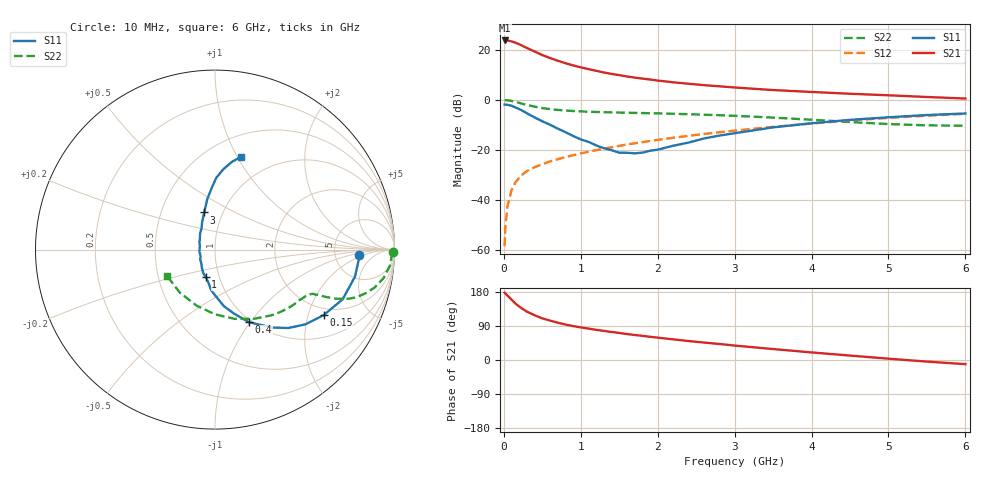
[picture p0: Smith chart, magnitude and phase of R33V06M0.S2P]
! SIEMENS Small Signal Semiconductors
! BFR181
! Si NPN RF Bipolar Junction Transistor in SOT23
! VCE = 3 V  IC = 6 mA
! Common Emitter S-Parameters:  May  1996
# GHz  S  MA  R  50
!  f  S11  S21  S12  S22
! GHz  MAG  ANG  MAG  ANG  MAG  ANG  MAG  ANG
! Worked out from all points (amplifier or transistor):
!   36 points, 10 MHz to 6 GHz, reference 50 ohm
!   highest |S21| = 23.7 dB at 10 MHz (marker M1)
!   |S21| within 3 dB of that: start of sweep to 300.1 MHz
!   unconditionally stable (mu >= 1): 993.5 MHz to 2.812 GHz
!   at 250 MHz: K = 0.47, MSG = 25.5 dB, |S12| = -29.6 dB
!   at 1.4 GHz: K = 1.05, MAG = 13.3 dB, |S12| = -18.9 dB
!   at 6 GHz: K = 0.86, MSG = 3.1 dB, |S12| = -5.6 dB
!   S11 on the Smith chart (normalised r, x): 10 MHz: 8.97, -1.65; 150 MHz: 1.73, -2.53; 400 MHz: 0.98, -0.99; 1 GHz: 0.86, -0.27; 3 GHz: 0.82, +0.36; 6 GHz: 0.71, +1.03
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0.01  0.8054 -2.3  15.34 177.7  0.0012 96.1  0.99 -0.9
0.02  0.8028 -4.1  15.31 175.4  0.003 88.9  0.9851 -2.0
0.05  0.7942 -11.0  15.33 169.3  0.0079 84.7  0.9804 -5.0
0.1  0.7631 -21.3  14.7 159.3  0.0157 80.6  0.9526 -9.6
0.15  0.707 -31.1  13.86 149.1  0.0225 74.4  0.9125 -13.5
0.2  0.6541 -39.5  12.9 141.1  0.0279 71.3  0.8698 -16.4
0.25  0.5983 -46.9  11.82 134.0  0.0332 68.2  0.8294 -18.7
0.3  0.5389 -53.7  10.86 127.7  0.0378 67.5  0.7933 -20.2
0.4  0.4469 -64.9  9.234 118.1  0.0453 65.2  0.731 -22.0
0.5  0.3732 -73.3  7.832 109.9  0.0519 64.8  0.6845 -22.9
0.6  0.3194 -81.0  6.846 104.0  0.059 64.4  0.6534 -23.4
0.8  0.2271 -95.5  5.397 93.7  0.0719 64.7  0.6135 -24.1
1  0.1621 -108.6  4.458 86.1  0.0853 65.6  0.5889 -24.9
1.1  0.1454 -116.9  4.11 82.9  0.0922 66.0  0.58 -25.5
1.3  0.1085 -134.3  3.522 76.9  0.1063 66.0  0.5674 -27.0
1.6  0.0878 -173.6  2.934 68.5  0.1285 65.6  0.554 -29.8
2.2  0.1213 133.4  2.242 54.5  0.175 63.6  0.5275 -37.1
3  0.2157 106.1  1.766 38.1  0.243 58.4  0.4802 -49.9
3.5  0.2824 98.9  1.57 28.9  0.289 54.2  0.4426 -60.5
4.5  0.3991 89.1  1.324 11.7  0.3877 43.8  0.3606 -90.0
5.5  0.498 79.1  1.141 -4.2  0.483 31.1  0.3095 -129.3
6  0.5354 74.5  1.063 -10.9  0.5265 24.0  0.3047 -150.9
